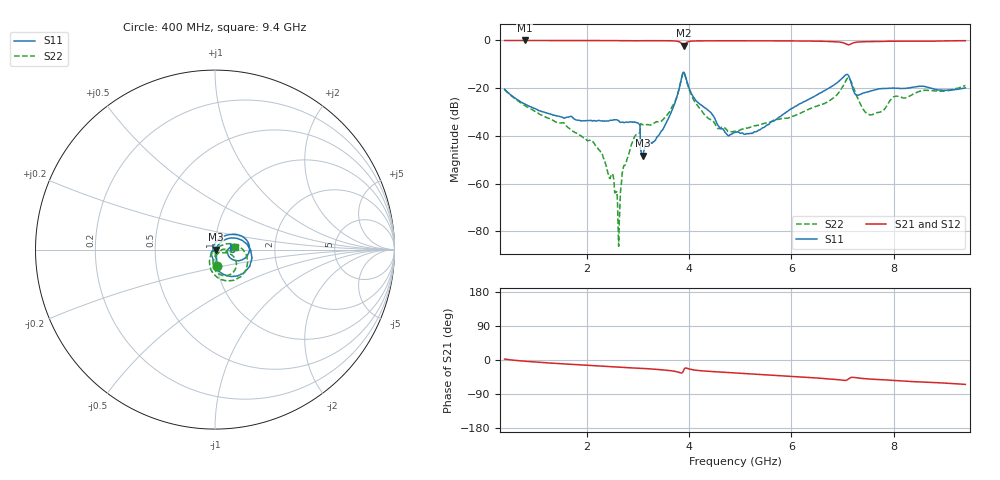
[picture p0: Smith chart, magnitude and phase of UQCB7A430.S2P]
!  Part Number  UQCB7A430	Mounting Orientation: Vertical
!  Description: RF capacitors
!  Application: Coupling, Bypass, Tuning, DC Block
!  Filters, Matching
# GHZ S DB R 50
! Freq  |S11|  S11 Ph  |S21|  S21 Ph  |S12|  S12 Ph  |S22|  S22 Ph
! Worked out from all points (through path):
!   801 points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, 400 MHz to 9.4 GHz, reference 50 ohm
!   highest |S21| = -0.10 dB at 794 MHz (marker M1); lowest = -2.3 dB at 3.899 GHz (marker M2)
!   group delay of S21, straight-line fit = 19.3 ps
!   lowest |S11| = -48.3 dB at 3.1 GHz (marker M3), VSWR 1.01, Z = 50.4 - j0.0902 ohm
!   |S11| at or under -10 dB: start of sweep to end of sweep
!   |S22| runs from -86.2 to -13.6 dB; largest |S21 - S12| = 0.0062
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0.4  -20.56 -81.9  -0.12 2.4  -0.08 2.4  -20.61 -83.6
0.794  -26.67 -80.0  -0.10 -3.2  -0.07 -3.2  -27.33 -85.1
1.908  -33.74 -64.5  -0.13 -13.1  -0.10 -13.1  -40.24 -88.2
2.29  -33.78 -61.1  -0.14 -16.2  -0.12 -16.3  -46.75 -96.5
2.538  -33.26 -61.0  -0.18 -18.2  -0.15 -18.3  -59.66 -85.7
2.616  -33.53 -65.7  -0.19 -18.7  -0.16 -18.8  -77.66 -91.2
2.74  -34.46 -61.5  -0.19 -19.7  -0.16 -19.8  -52.40 94.7
2.999  -34.63 -67.6  -0.25 -21.5  -0.22 -21.6  -39.34 71.8
3.1  -48.26 -13.4  -0.21 -22.1  -0.18 -22.2  -35.28 32.4
3.404  -39.99 37.9  -0.17 -25.1  -0.15 -25.2  -34.14 27.2
3.663  -29.63 55.1  -0.24 -28.5  -0.21 -28.6  -28.18 33.9
3.899  -13.36 -26.0  -2.31 -26.4  -2.29 -26.5  -13.59 -45.5
4.326  -28.46 -119.5  -0.27 -29.3  -0.25 -29.5  -31.61 -129.9
4.743  -39.38 -141.1  -0.22 -32.7  -0.20 -32.9  -37.52 -111.3
4.9  -38.56 -137.3  -0.19 -34.2  -0.18 -34.4  -38.14 -89.8
5.339  -38.00 155.9  -0.24 -38.0  -0.23 -38.1  -35.62 -65.4
6.408  -23.97 68.4  -0.36 -46.6  -0.37 -46.9  -28.27 -26.5
7.105  -14.48 -5.8  -1.88 -51.1  -1.89 -51.4  -15.81 -51.1
7.263  -22.88 -13.9  -0.86 -46.8  -0.87 -47.0  -22.54 -98.5
7.499  -21.57 7.0  -0.58 -49.9  -0.60 -50.2  -30.98 -63.5
7.904  -20.12 2.0  -0.43 -53.1  -0.44 -53.4  -25.99 2.9
9.4  -19.96 7.8  -0.20 -64.4  -0.23 -64.6  -18.96 7.2
